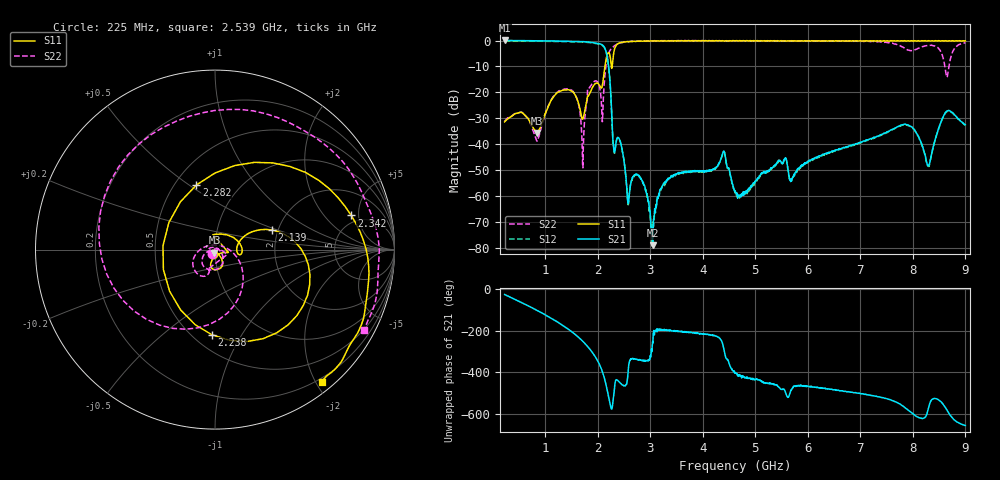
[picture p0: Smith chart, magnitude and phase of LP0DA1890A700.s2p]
!Agilent Technologies,E8358A,US41080443,A.07.50.56
!Agilent E8358A: A.07.50.56
!Date: Wednesday, August 31, 2016 09:27:32
!Correction: S11(Full 2 Port(1,2))
!S21(Full 2 Port(1,2))
!S12(Full 2 Port(1,2))
!S22(Full 2 Port(1,2))
!S2P File: Measurements: S11, S21, S12, S22:
# Hz S  dB  R 50
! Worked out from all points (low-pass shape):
!   1601 points, 225 MHz to 9 GHz, reference 50 ohm
!   highest |S21| = 0.06 dB at 225 MHz (marker M1); lowest = -79.1 dB at 3.044 GHz (marker M2)
!   |S21| within 3 dB of the highest: start of sweep to 2.134 GHz
!   lowest |S11| = -35.6 dB at 833.8 MHz (marker M3), VSWR 1.03, Z = 49.7 - j1.62 ohm
!   |S11| at or under -10 dB: start of sweep to 2.136 GHz; 2.258 GHz to 2.274 GHz (15.59 MHz wide, 0.688 % of centre)
!   |S22| runs from -49.1 to 0.0 dB; largest |S21 - S12| = 0.023
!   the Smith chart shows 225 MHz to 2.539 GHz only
!   S11 on the Smith chart (normalised r, x): 225 MHz: 0.98, -0.05; 2.139 GHz: 1.85, +0.46; 2.238 GHz: 0.62, -0.76; 2.282 GHz: 0.64, +0.53; 2.342 GHz: 4.11, +4.03; 2.539 GHz: 0.15, -2.09
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2.25e8  -31.40 -110.9  0.06 -26.7  -0.13 -26.4  -31.16 -123.9
8.337656e8  -35.64 -99.9  -0.04 -101.5  -0.23 -101.2  -38.59 80.4
1.36575e9  -19.06 -81.5  -0.23 179.5  -0.41 179.8  -18.74 -99.7
1.689328e9  -29.41 -85.1  -0.38 114.5  -0.55 114.8  -34.17 -176.8
1.996453e9  -16.47 -7.2  -1.06 14.8  -1.25 15.2  -15.98 -137.8
2.139047e9  -9.51 19.1  -3.17 -82.5  -3.35 -82.1  -12.53 -48.3
2.237766e9  -6.46 -91.9  -17.49 161.3  -17.70 161.9  -3.62 169.1
2.281641e9  -8.53 106.0  -36.80 164.1  -36.94 164.3  -2.62 112.7
2.341969e9  -2.13 14.1  -39.95 -79.3  -40.14 -79.3  -1.69 56.5
2.539406e9  -0.47 -50.9  -53.53 -99.7  -54.06 -100.5  -0.50 -28.4
3.043969e9  -0.22 -95.6  -79.14 107.4  -72.50 77.0  -0.11 -89.5
3.153656e9  -0.13 -100.9  -60.16 163.0  -60.15 159.5  -0.06 -96.1
4.387641e9  -0.06 -129.7  -42.98 85.6  -43.17 87.0  -0.09 -144.6
4.6125e9  -0.12 -132.4  -58.04 -43.9  -57.93 -45.9  -0.07 -152.4
6.076828e9  -0.04 -158.5  -45.80 -110.1  -46.23 -110.6  -0.18 130.9
7.541156e9  -0.19 173.9  -35.03 -170.8  -35.12 -170.5  -0.83 35.7
7.947e9  -0.15 169.4  -33.07 130.7  -33.19 130.5  -3.87 -89.4
8.133469e9  -0.19 166.8  -38.28 99.6  -38.49 99.1  -2.76 -178.8
8.374781e9  -0.06 163.6  -42.02 -169.4  -42.25 -168.9  -1.93 115.1
8.572219e9  -0.08 162.0  -29.53 166.6  -29.73 167.5  -6.44 46.8
8.687391e9  -0.06 161.2  -26.97 121.9  -27.20 122.2  -9.94 -126.3
9e9  -0.09 158.3  -32.46 63.7  -32.64 63.5  -0.77 134.8
